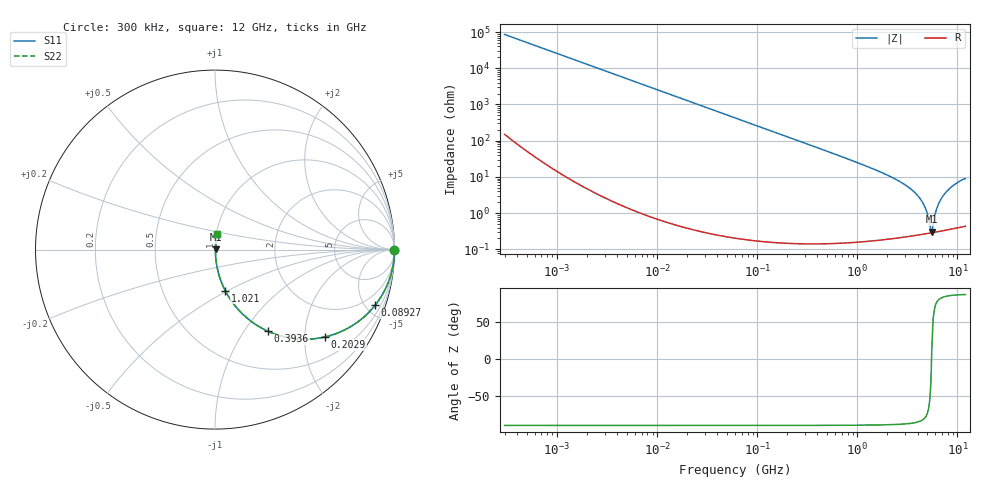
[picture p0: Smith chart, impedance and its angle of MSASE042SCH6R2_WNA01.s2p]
! MSASE042SCH6R2_WNA01  S-PARAMETER MODEL  ( General Type )
! Model Generated by TAIYO YUDEN Corporation (http://www.ty-top.com)
! Version 1.0
! TAIYO YUDEN Control No. 120810
! Copyright(c) 2012 TAIYO YUDEN CO.,LTD. All Rights Reserved.
! Product Description (link to TY-COMPAS)
! https://ds.yuden.co.jp/TYCOMPAS/or/detail?pn=MSASE042SCH6R2BWNA01&u=M
! Products Name : Multilayer Ceramic Capacitors
! Characteristics :
!  Capacitance : 6.2 pF , Rated Voltage : 16V , TCC : CH / C0H
!  Case Size : 0.4 x 0.2 / 0.016 x 0.008 [mm/inch] , Thickness : 0.2 / 0.008 [mm/inch]
!  (Conditions: Temperature = 25 degC , DC Bias Current/Voltage = 0A / 0V)
! External Node Assignments :
!  1  o---| |---o  2
! GND o---------o GND
! Frequency Range : 0.3MHz  -  12000MHz  [ 401 STEP ]
# MHz S RI R 50
! Freq[MHz].  S11 Real  S11 Imag  S21 Real  S21 Imag  S12 Real  S12 Imag  S22 Real  S22 Imag
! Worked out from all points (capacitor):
!   401 points, 300 kHz to 12 GHz, reference 50 ohm
!   read as one part in series: C = 6.21 pF near 316.3 kHz
!   lowest |Z| = 306 mohm at 5.566 GHz (marker M1)
!   series resonance near 5.513 GHz, so ESL is about 130 pH
!   S11 on the Smith chart (normalised r, x): 300 kHz: open; 89.27 MHz: 1.00, -5.74; 202.9 MHz: 1.00, -2.52; 393.6 MHz: 1.00, -1.30; 1.021 GHz: 1.00, -0.48; 12 GHz: 1.01, +0.18
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0.3  1 -0.00117  3.41e-06 0.00117  3.41e-06 0.00117  1 -0.00117
1.769972  0.9999 -0.0069  5.03e-05 0.0069  5.03e-05 0.0069  0.9999 -0.0069
10.44266  0.9983 -0.0407  0.00167 0.0407  0.00167 0.0407  0.9983 -0.0407
60  0.948 -0.2218  0.052 0.2218  0.052 0.2218  0.948 -0.2218
89.27472  0.8917 -0.3104  0.1083 0.3104  0.1083 0.3104  0.8917 -0.3104
202.9496  0.6141 -0.4862  0.3859 0.4862  0.3859 0.4862  0.6141 -0.4862
353.9943  0.3426 -0.4736  0.6574 0.4736  0.6574 0.4736  0.3426 -0.4736
393.5654  0.2963 -0.4555  0.7037 0.4555  0.7037 0.4555  0.2963 -0.4555
617.4538  0.1449 -0.3502  0.8551 0.3502  0.8551 0.3502  0.1449 -0.3502
1021.415  0.0569 -0.2283  0.9431 0.2283  0.9431 0.2283  0.0569 -0.2283
2088.533  0.0128 -0.1037  0.9872 0.1037  0.9872 0.1037  0.0128 -0.1037
3026.31  0.00568 -0.0589  0.9943 0.0589  0.9943 0.0589  0.00568 -0.0589
3944.255  0.00345 -0.0317  0.9965 0.0317  0.9965 0.0317  0.00345 -0.0317
4623.766  0.0029 -0.0166  0.9971 0.0166  0.9971 0.0166  0.0029 -0.0166
4875.354  0.00282 -0.0116  0.9972 0.0116  0.9972 0.0116  0.00282 -0.0116
5278.635  0.00281 -0.00426  0.9972 0.00426  0.9972 0.00426  0.00281 -0.00426
5565.855  0.00286 0.00106  0.9971 -0.00106  0.9971 -0.00106  0.00286 0.00106
5715.274  0.00292 0.00405  0.9971 -0.00405  0.9971 -0.00405  0.00292 0.00405
6354.153  0.00329 0.0154  0.9967 -0.0154  0.9967 -0.0154  0.00329 0.0154
7254.098  0.00422 0.0307  0.9958 -0.0307  0.9958 -0.0307  0.00422 0.0307
8966.534  0.0068 0.0559  0.9932 -0.0559  0.9932 -0.0559  0.0068 0.0559
12000  0.0122 0.0883  0.9878 -0.0883  0.9878 -0.0883  0.0122 0.0883
